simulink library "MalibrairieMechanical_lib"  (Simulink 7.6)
settings: Solver=ode45  StartTime=0.0  StopTime=10.0  RelTol=1e-3
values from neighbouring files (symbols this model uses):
  m = 10    [masse_ressort_enveloppe.m]
  N = 50;')    [Prog_callbacks.m]    (also in _startup.m = 0.001'))
undefined symbols (not defined in the file or in its folder): gcbh, MalibrairieMechanical, nesl_callback, Ressort_NLs, spring

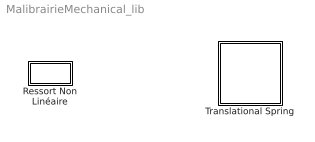
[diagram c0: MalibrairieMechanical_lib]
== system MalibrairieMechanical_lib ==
  Ressort Non Linéaire : Subsystem  DialogController=NetworkEngine.DynNeDlgSource  LoadFcn=nesl_callback('LoadFcn',gcbh);  mask(Ressort Non Linéaire){ComponentPath=MalibrairieMechanical.Ressort_NL, ClassName=Ressort_NLs, SchemaVersion=1, k1=500, k1_unit=N/m, k2=1000, k2_unit=N/m, l=0.1, l_unit=m, x0=0, x0_unit=m, f_Log=off, v_Log=off, x_Log=off, k_Log=off, LocalVarNames=\, LocalVarDescs=f\, LocalVarLogging=v\}
      mask prompts: k1 "raideur1"; k2 "raideur2"; l "longueur du ressort"; x0 "longueur du ressort"
      mask init:
      | nesl_preinitmask (gcb);
  Translational Spring : Subsystem  DialogController=NetworkEngine.DynNeDlgSource  LoadFcn=nesl_callback('LoadFcn',gcbh);  mask(Translational Spring){ComponentPath=MalibrairieMechanical.R_NL2, ClassName=spring, SchemaVersion=1, k1=500, k1_unit=N/m, k2=1000, k2_unit=N/m, x0=0, x0_unit=m, f_Log=off, v_Log=off, k_Log=off, x_Log=off, LocalVarNames=\, LocalVarDescs=f\, LocalVarLogging=v\}
      mask prompts: k1 "Spring rate"; k2 "Spring rate"; x0 "Initial deformation"
      mask help: The block represents an ideal mechanical linear spring. Connections R and C are mechanical translational conserving ports. The block positive direction is from port R to port C. This means that the force is positive if it acts in the direction from R to C.
      mask init:
      | nesl_preinitmask (gcb);

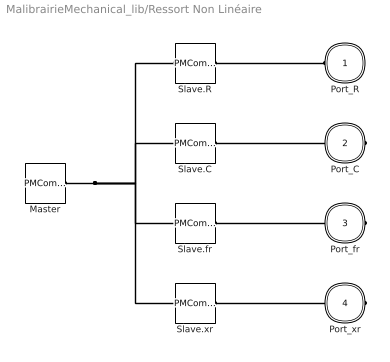
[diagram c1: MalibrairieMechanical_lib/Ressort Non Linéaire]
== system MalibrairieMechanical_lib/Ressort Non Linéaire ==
  Master : PMComponent  Tag=MalibrairieMechanical.Ressort_NL  PhysicalDomain=network_engine_domain  SubClassName=master  LeftPortType=generic  RightPortType=generic  RConnTagsString=RConn1
  Slave.C : PMComponent  Tag=C  PhysicalDomain=network_engine_domain  SubClassName=terminal  LeftPortType=generic  RightPortType=foundation.mechanical.translational.translational  LConnTagsString=LConn1  RConnTagsString=RConn1
  Slave.R : PMComponent  Tag=R  PhysicalDomain=network_engine_domain  SubClassName=terminal  LeftPortType=generic  RightPortType=foundation.mechanical.translational.translational  LConnTagsString=LConn1  RConnTagsString=RConn1
  Slave.fr : PMComponent  Tag=fr  PhysicalDomain=network_engine_domain  SubClassName=output  LeftPortType=generic  RightPortType=output  LConnTagsString=LConn1  RConnTagsString=RConn1
  Slave.xr : PMComponent  Tag=xr  PhysicalDomain=network_engine_domain  SubClassName=output  LeftPortType=generic  RightPortType=output  LConnTagsString=LConn1  RConnTagsString=RConn1
  Port_R : PMIOPort  Tag=R  Port=1  Side=Left
  Port_C : PMIOPort  Tag=C  Port=2  Side=Right
  Port_fr : PMIOPort  Tag=fr  Port=3  Side=Right
  Port_xr : PMIOPort  Tag=xr  Port=4  Side=Right
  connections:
  Slave.R/RConn1 -- Port_R/RConn1
  Slave.R/LConn1 -- Slave.C/LConn1 -- Slave.fr/LConn1 -- Master/RConn1 -- Slave.xr/LConn1
  Slave.C/RConn1 -- Port_C/RConn1
  Slave.fr/RConn1 -- Port_fr/RConn1
  Slave.xr/RConn1 -- Port_xr/RConn1

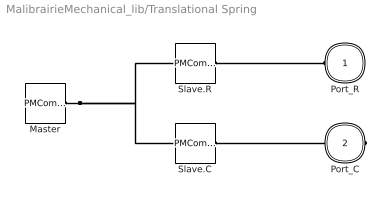
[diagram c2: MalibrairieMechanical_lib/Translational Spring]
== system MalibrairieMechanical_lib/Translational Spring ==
  Master : PMComponent  Tag=MalibrairieMechanical.R_NL2  PhysicalDomain=network_engine_domain  SubClassName=master  LeftPortType=generic  RightPortType=generic  RConnTagsString=RConn1
  Slave.C : PMComponent  Tag=C  PhysicalDomain=network_engine_domain  SubClassName=terminal  LeftPortType=generic  RightPortType=foundation.mechanical.translational.translational  LConnTagsString=LConn1  RConnTagsString=RConn1
  Slave.R : PMComponent  Tag=R  PhysicalDomain=network_engine_domain  SubClassName=terminal  LeftPortType=generic  RightPortType=foundation.mechanical.translational.translational  LConnTagsString=LConn1  RConnTagsString=RConn1
  Port_R : PMIOPort  Tag=R  Port=1  Side=Left
  Port_C : PMIOPort  Tag=C  Port=2  Side=Right
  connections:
  Slave.R/RConn1 -- Port_R/RConn1
  Master/RConn1 -- Slave.R/LConn1 -- Slave.C/LConn1
  Slave.C/RConn1 -- Port_C/RConn1
